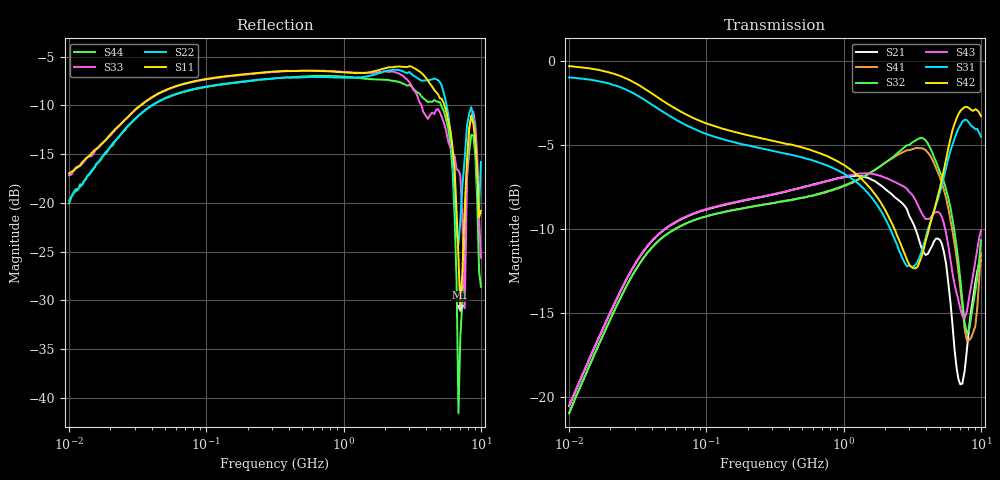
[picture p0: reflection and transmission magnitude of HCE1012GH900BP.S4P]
!Agilent Technologies,E5071C,MY46111244,A.11.31
!Date: Tue May 14 17:30:54 2019
!Data & Calibration Information:
!Freq	S11:SOLT4(ON)	S12:SOLT4(ON)	S13:SOLT4(ON)	S14:SOLT4(ON)
!	S21:SOLT4(ON)	S22:SOLT4(ON)	S23:SOLT4(ON)	S24:SOLT4(ON)
!	S31:SOLT4(ON)	S32:SOLT4(ON)	S33:SOLT4(ON)	S34:SOLT4(ON)
!	S41:SOLT4(ON)	S42:SOLT4(ON)	S43:SOLT4(ON)	S44:SOLT4(ON)
!PortZ  Port1:50+j0  Port2:50+j0  Port3:50+j0  Port4:50+j0
!Above PortZ is port z conversion or system Z0 setting when saving the data.
!When reading, reference impedance value at option line is always used.
# Hz S dB R 50
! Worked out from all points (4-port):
!   201 points, 10 MHz to 10 GHz, reference 50 ohm
!   strongest paths, dB at 10 MHz, 56.66 MHz, 319.3 MHz, 1.79 GHz, 10 GHz:
!     S42: -0.3, -2.7, -4.8, -8.2, -3.3
!     S31: -1.0, -3.4, -5.4, -8.7, -4.5
!     S43: -20.5, -9.7, -7.9, -6.8, -10.1
!     S32: -21.0, -10.1, -8.4, -6.3, -10.7
!     S41: -21.0, -10.1, -8.4, -6.3, -11.4
!     S21: -20.6, -9.7, -7.9, -7.3, -11.9
!   lowest |S11| = -30.7 dB at 7.079 GHz (marker M1), VSWR 1.06, Z = 47.7 - j1.67 ohm
!   |S11| at or under -10 dB: start of sweep to 33.1 MHz; 5.428 GHz to end of sweep
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1e7  -16.98 40.3  -20.55 78.2  -0.95 -6.1  -20.93 -102.4
     -20.56 78.1  -19.74 66.8  -20.98 -102.4  -0.30 -6.0
     -0.96 -6.0  -20.99 -102.4  -17.16 39.9  -20.51 78.1
     -20.98 -102.3  -0.28 -6.0  -20.53 78.0  -20.04 68.9
3.007797e9  -5.97 -29.6  -9.14 -29.3  -12.16 -175.1  -5.28 25.4
            -9.22 -29.4  -6.57 -25.9  -4.98 26.7  -12.21 -166.4
            -12.17 -175.7  -4.98 26.5  -7.61 -32.8  -7.75 -23.0
            -5.29 25.5  -12.12 -166.7  -7.78 -23.1  -7.90 -29.1
5.797603e9  -11.70 -96.1  -13.23 -48.9  -5.77 20.5  -8.74 -64.8
            -13.25 -47.9  -11.00 -98.2  -8.15 -64.4  -5.22 20.3
            -5.77 20.2  -8.17 -64.2  -13.79 -76.6  -10.99 -44.5
            -8.77 -64.3  -5.16 19.9  -11.01 -43.9  -12.47 -101.4
7.079458e9  -30.73 -143.0  -19.23 -19.0  -3.80 -22.9  -13.69 -84.1
            -19.26 -20.8  -21.86 172.8  -12.95 -85.9  -2.95 -24.9
            -3.82 -23.1  -12.97 -86.1  -17.11 -3.2  -14.73 -33.7
            -13.48 -84.0  -2.96 -25.2  -14.75 -34.9  -33.83 18.8
7.625107e9  -20.55 -151.7  -18.32 -0.6  -3.45 -41.5  -16.14 -79.0
            -18.44 -2.2  -15.43 -176.7  -15.69 -81.0  -2.75 -42.7
            -3.48 -41.4  -15.63 -81.4  -30.81 -105.9  -15.21 -25.0
            -15.96 -79.8  -2.72 -42.7  -15.29 -24.8  -24.77 -108.2
8.515692e9  -11.03 -157.4  -14.81 0.8  -3.87 -68.2  -16.20 -59.0
            -14.77 1.7  -10.18 -155.3  -15.35 -56.6  -2.98 -68.1
            -3.85 -68.3  -15.20 -57.1  -11.12 -151.0  -13.45 -18.7
            -16.46 -59.3  -2.90 -68.2  -13.35 -17.7  -13.01 -156.8
1e10  -20.82 120.1  -11.78 -23.0  -4.45 -108.1  -11.46 -43.2
      -11.87 -24.7  -15.79 84.7  -10.55 -53.6  -3.30 -107.7
      -4.47 -108.0  -10.67 -53.7  -25.62 127.4  -10.08 -40.7
      -11.43 -43.2  -3.26 -107.9  -10.09 -40.9  -28.59 145.0
